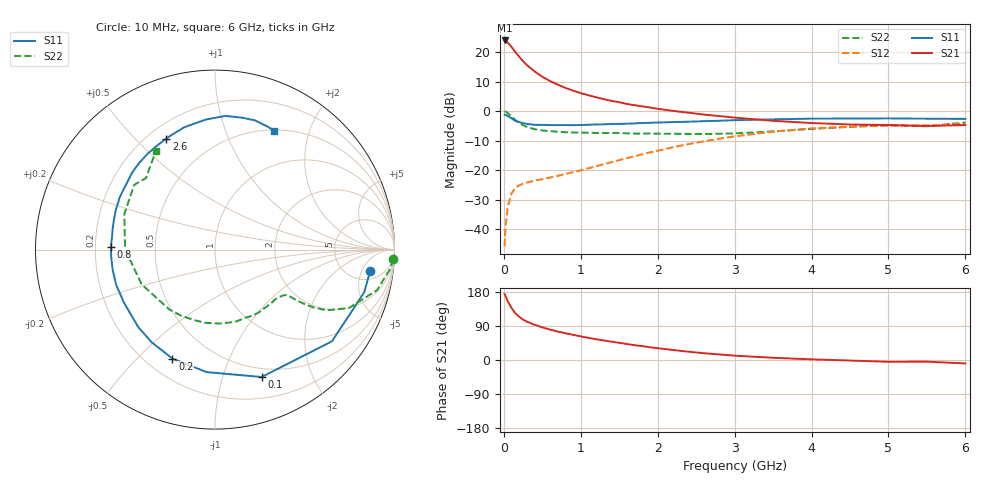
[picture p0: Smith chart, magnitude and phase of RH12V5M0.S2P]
! SIEMENS Small Signal Semiconductors
! BFR106
! Si NPN RF Bipolar Junction Transistor in SOT23
! VCE = 12 V  IC = 5 mA
! Common Emitter S-Parameters:  August  1996
# GHz  S  MA  R  50
!  f  S11  S21  S12  S22
! GHz  MAG  ANG  MAG  ANG  MAG  ANG  MAG  ANG
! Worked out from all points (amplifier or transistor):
!   36 points, 10 MHz to 6 GHz, reference 50 ohm
!   highest |S21| = 24.0 dB at 10 MHz (marker M1)
!   |S21| within 3 dB of that: start of sweep to 122.7 MHz
!   unconditionally stable (mu >= 1): 636.1 MHz to 1.84 GHz; 5.054 GHz to end of sweep
!   at 250 MHz: K = 0.50, MSG = 20.8 dB, |S12| = -24.6 dB
!   at 1.4 GHz: K = 1.13, MAG = 8.2 dB, |S12| = -17.3 dB
!   at 6 GHz: K = 1.02, MAG = -1.0 dB, |S12| = -4.3 dB
!   S11 on the Smith chart (normalised r, x): 10 MHz: 7, -7; 100 MHz: 0.41, -1.35; 200 MHz: 0.30, -0.64; 800 MHz: 0.27, +0.01; 2.6 GHz: 0.27, +0.62; 6 GHz: 0.51, +1.49
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0.01  0.8724 -8.0  15.88 174.2  0.0051 87.4  0.9925 -3.1
0.02  0.8646 -16.0  15.77 169.8  0.0104 81.4  0.9846 -6.0
0.05  0.8281 -38.1  14.63 155.3  0.0235 70.2  0.9301 -14.1
0.1  0.7559 -69.9  12.32 137.3  0.0405 57.0  0.8138 -23.6
0.15  0.6841 -93.9  10.07 123.0  0.0494 47.9  0.7068 -28.6
0.2  0.652 -111.3  8.392 114.0  0.0549 44.2  0.6324 -30.5
0.25  0.6254 -124.3  7.046 106.5  0.059 41.1  0.5758 -31.4
0.3  0.6077 -134.7  6.057 101.2  0.0615 40.7  0.541 -31.8
0.4  0.587 -149.8  4.728 92.9  0.066 41.1  0.4941 -32.0
0.5  0.5846 -160.4  3.836 86.0  0.07 42.9  0.4696 -32.6
0.6  0.5811 -169.1  3.253 80.3  0.0747 45.9  0.4574 -34.0
0.8  0.5807 178.4  2.489 70.7  0.0857 51.7  0.4397 -37.8
1.1  0.5879 163.0  1.86 58.5  0.1073 59.5  0.43 -45.7
1.3  0.5986 155.1  1.598 51.5  0.1258 62.9  0.4258 -51.7
1.6  0.6131 144.1  1.326 42.1  0.1594 65.7  0.4207 -62.0
2.2  0.6523 125.4  1.011 26.3  0.2441 64.1  0.4127 -86.4
2.6  0.6759 113.7  0.875 17.9  0.3074 59.1  0.4099 -106.0
3.5  0.7267 93.9  0.686 5.9  0.4501 43.1  0.4521 -154.6
4.5  0.7502 78.6  0.594 -1.4  0.546 22.6  0.5424 158.7
5  0.7537 72.9  0.582 -4.8  0.5689 13.9  0.5772 141.3
5.5  0.7454 67.0  0.56 -4.4  0.573 9.3  0.5536 134.0
6  0.7408 63.6  0.581 -9.1  0.6088 1.0  0.6419 120.8
